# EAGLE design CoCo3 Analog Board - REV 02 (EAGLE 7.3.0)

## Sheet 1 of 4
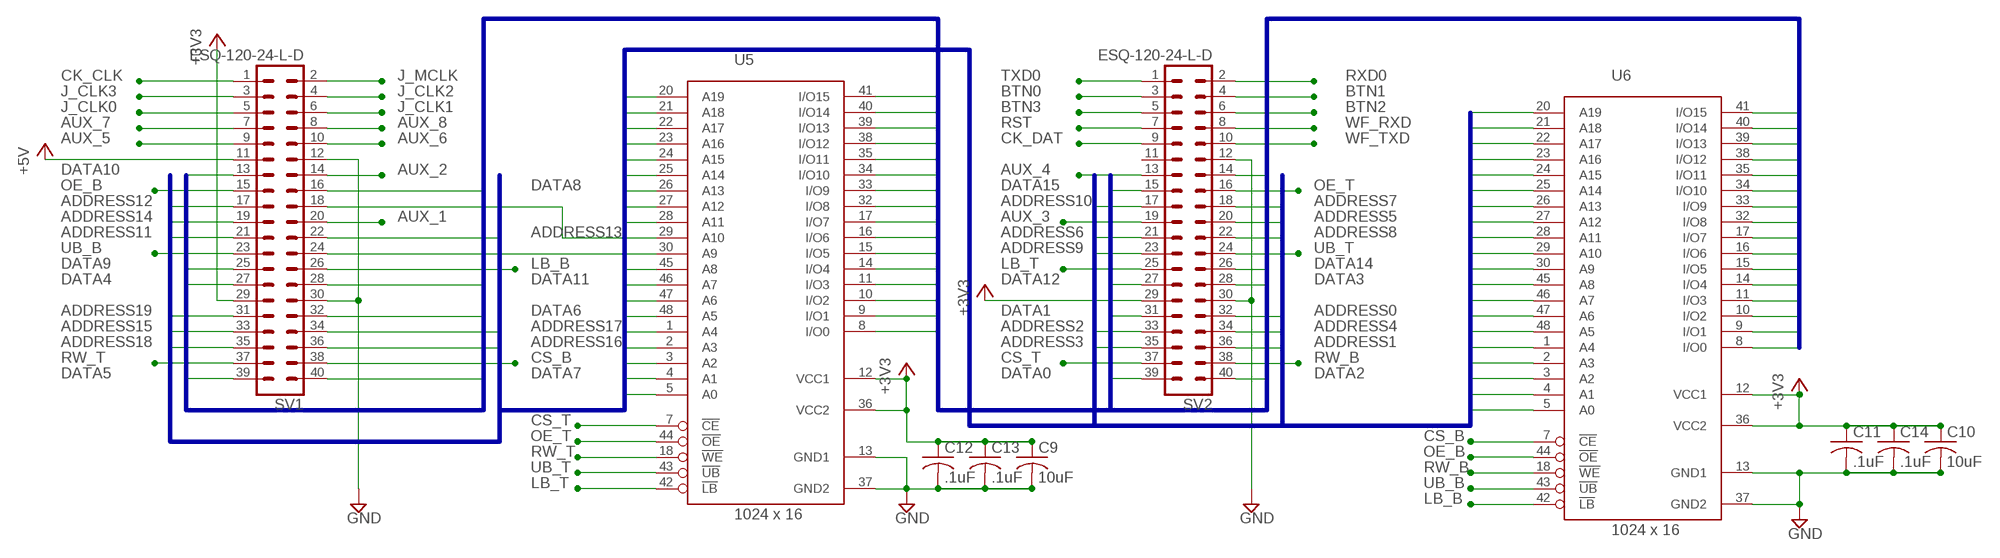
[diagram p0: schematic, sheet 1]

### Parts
C9  10uF  C-USC0805  [C0805]
C10  10uF  C-USC0805  [C0805]
C11  .1uF  C-USC0603  [C0603]
C12  .1uF  C-USC0603  [C0603]
C13  .1uF  C-USC0603  [C0603]
C14  .1uF  C-USC0603  [C0603]
SV1  ESQ-120-24-L-D  MA20-2  [MA20-2]
SV2  ESQ-120-24-L-D  MA20-2  [MA20-2]
U5  1024 x 16  IS62WV102416BLL-25T  [TSOP-I-48-12X40MM]
U6  1024 x 16  IS62WV102416BLL-25T  [TSOP-I-48-12X40MM]

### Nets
+3V3: C9.1 C10.1 C11.1 C12.1 C13.1 C14.1 SV1.29 SV2.29 U5.12(VCC1) U5.36(VCC2) U6.12(VCC1) U6.36(VCC2) ; also sheet 2,4
+5V: SV1.11 ; also sheet 3,4
ADDRESS0: SV2.32 U5.5(A0) U6.20(A19)
ADDRESS1: SV2.36 U5.4(A1) U6.21(A18)
ADDRESS2: SV2.33 U5.3(A2) U6.22(A17)
ADDRESS3: SV2.35 U5.2(A3) U6.23(A16)
ADDRESS4: SV2.34 U5.1(A4) U6.24(A15)
ADDRESS5: SV2.20 U5.48(A5) U6.25(A14)
ADDRESS6: SV2.21 U5.47(A6) U6.26(A13)
ADDRESS7: SV2.18 U5.46(A7) U6.27(A12)
ADDRESS8: SV2.22 U5.45(A8) U6.28(A11)
ADDRESS9: SV2.23 U6.30(A9)
ADDRESS9T: SV1.24 U5.30(A9)
ADDRESS10: SV2.17 U6.29(A10)
ADDRESS10T: SV1.18 U5.29(A10)
ADDRESS11: SV1.21 U5.28(A11) U6.45(A8)
ADDRESS12: SV1.17 U5.27(A12) U6.46(A7)
ADDRESS13: SV1.22 U5.26(A13) U6.47(A6)
ADDRESS14: SV1.19 U5.25(A14) U6.48(A5)
ADDRESS15: SV1.33 U5.24(A15) U6.1(A4)
ADDRESS16: SV1.36 U5.23(A16) U6.2(A3)
ADDRESS17: SV1.34 U5.22(A17) U6.3(A2)
ADDRESS18: SV1.35 U5.21(A18) U6.4(A1)
ADDRESS19: SV1.31 U5.20(A19) U6.5(A0)
AUX_1: SV1.20 ; also sheet 4
AUX_2: SV1.14 ; also sheet 4
AUX_3: SV2.19 ; also sheet 4
AUX_4: SV2.13 ; also sheet 4
AUX_5: SV1.9 ; also sheet 4
AUX_6: SV1.10 ; also sheet 4
AUX_7: SV1.7 ; also sheet 4
AUX_8: SV1.8 ; also sheet 4
BTN0: SV2.3 ; also sheet 3
BTN1: SV2.4 ; also sheet 3
BTN2: SV2.6 ; also sheet 3
BTN3: SV2.5 ; also sheet 3
CK_CLK: SV1.1 ; also sheet 4
CK_DAT: SV2.9 ; also sheet 4
CS_B: SV1.38 U6.7(!CE)
CS_T: SV2.37 U5.7(!CE)
DATA0: SV2.39 U5.8(I/O0) U6.17(I/O7)
DATA1: SV2.31 U5.9(I/O1) U6.16(I/O6)
DATA2: SV2.40 U5.10(I/O2) U6.15(I/O5)
DATA3: SV2.28 U5.11(I/O3) U6.14(I/O4)
DATA4: SV1.27 U5.14(I/O4) U6.11(I/O3)
DATA5: SV1.39 U5.15(I/O5) U6.10(I/O2)
DATA6: SV1.32 U5.16(I/O6) U6.9(I/O1)
DATA7: SV1.40 U5.17(I/O7) U6.8(I/O0)
DATA8: SV1.16 U5.32(I/O8) U6.41(I/O15)
DATA9: SV1.25 U5.33(I/O9) U6.40(I/O14)
DATA10: SV1.13 U5.34(I/O10) U6.39(I/O13)
DATA11: SV1.28 U5.35(I/O11) U6.38(I/O12)
DATA12: SV2.27 U5.38(I/O12) U6.35(I/O11)
DATA13: SV2.14 U5.39(I/O13) U6.34(I/O10)
DATA14: SV2.26 U5.40(I/O14) U6.33(I/O9)
DATA15: SV2.15 U5.41(I/O15) U6.32(I/O8)
GND: C9.2 C10.2 C11.2 C12.2 C13.2 C14.2 SV1.12 SV1.30 SV2.12 SV2.30 U5.13(GND1) U5.37(GND2) U6.13(GND1) U6.37(GND2) ; also sheet 2,3,4
J_CLK0: SV1.5 ; also sheet 3
J_CLK1: SV1.6 ; also sheet 3
J_CLK2: SV1.4 ; also sheet 3
J_CLK3: SV1.3 ; also sheet 3
J_MCLK: SV1.2 ; also sheet 3
LB_B: SV1.26 U6.42(!LB)
LB_T: SV2.25 U5.42(!LB)
OE_B: SV1.15 U6.44(!OE)
OE_T: SV2.16 U5.44(!OE)
RST: SV2.7 ; also sheet 4
RW_B: SV2.38 U6.18(!WE)
RW_T: SV1.37 U5.18(!WE)
RXD0: SV2.2 ; also sheet 2
TXD0: SV2.1 ; also sheet 2
UB_B: SV1.23 U6.43(!UB)
UB_T: SV2.24 U5.43(!UB)
WF_RXD: SV2.8 ; also sheet 4
WF_TXD: SV2.10 ; also sheet 4
Unconnected: SV2.11

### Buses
DATA[0..15]
ADDRESS[0..19]

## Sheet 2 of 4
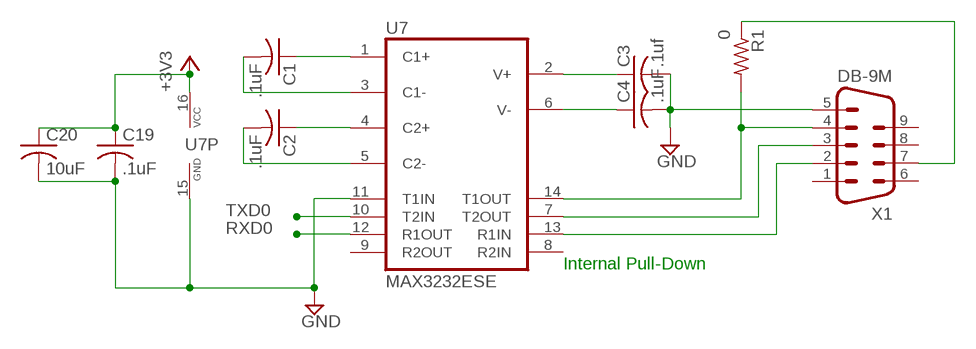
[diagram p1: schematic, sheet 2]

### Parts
C1  .1uF  C-USC0603  [C0603]
C2  .1uF  C-USC0603  [C0603]
C3  .1uf  C-USC0603  [C0603]
C4  .1uF  C-USC0603  [C0603]
C19  .1uF  C-USC0603  [C0603]
C20  10uF  C-USC0805  [C0805]
R1  0  R-US_M0805  [M0805]
U7  MAX3232ESE  [SO16]
X1  DB-9M  M09HP  [M09HP]

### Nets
+3V3: C19.1 C20.1 U7.16(VCC) ; also sheet 1,4
GND: C3.2 C4.2 C19.2 C20.2 U7.11(T1IN) U7.15(GND) X1.5 ; also sheet 1,3,4
N$1: C1.1 U7.1(C1+)
N$2: C1.2 U7.3(C1-)
N$3: C2.1 U7.4(C2+)
N$4: C2.2 U7.5(C2-)
N$5: C3.1 U7.2(V+)
N$6: C4.1 U7.6(V-)
N$8: U7.13(R1IN) X1.2
N$9: U7.7(T2OUT) X1.3
N$27: R1.1 X1.7
N$28: R1.2 U7.14(T1OUT) X1.4
RXD0: U7.12(R1OUT) ; also sheet 1
TXD0: U7.10(T2IN) ; also sheet 1
Unconnected: U7.8(R2IN) U7.9(R2OUT) X1.1 X1.6 X1.8 X1.9

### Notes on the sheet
- Internal Pull-Down

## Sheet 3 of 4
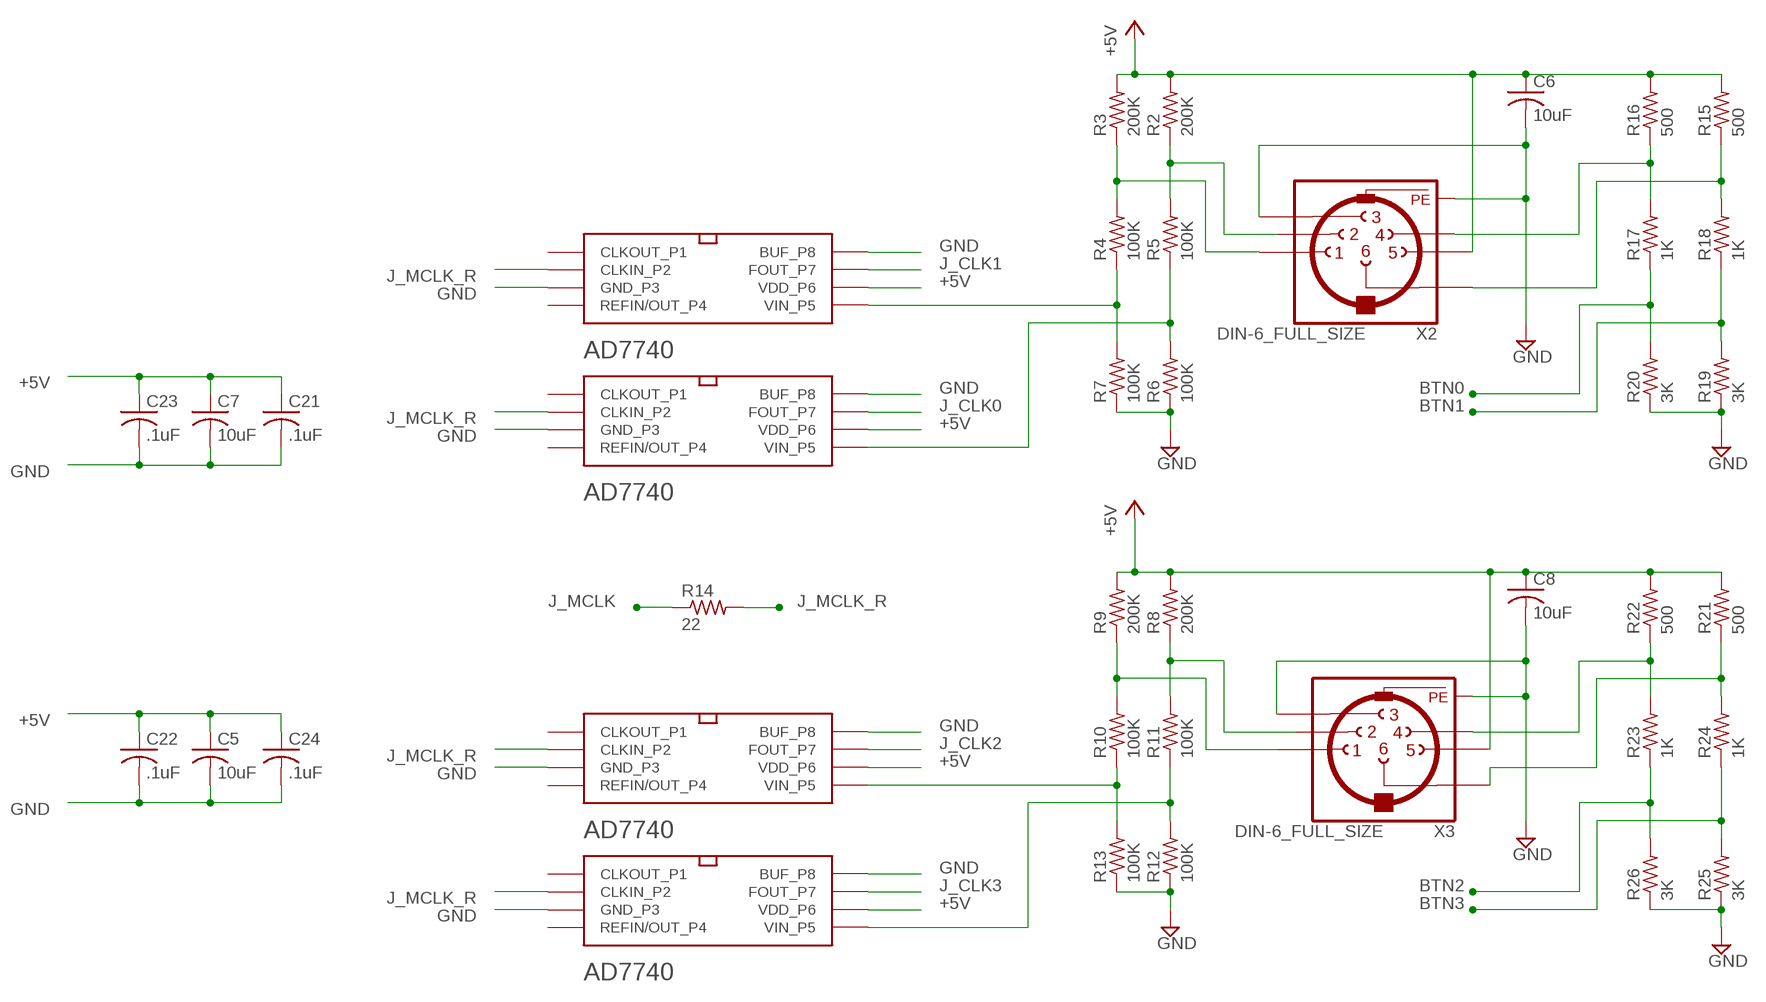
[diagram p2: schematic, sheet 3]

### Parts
C5  10uF  C-USC0805K  [C0805K]
C6  10uF  C-USC0805K  [C0805K]
C7  10uF  C-USC0805K  [C0805K]
C8  10uF  C-USC0805K  [C0805K]
C21  .1uF  C-USC0603  [C0603]
C22  .1uF  C-USC0603  [C0603]
C23  .1uF  C-USC0603  [C0603]
C24  .1uF  C-USC0603  [C0603]
R2  200K  R-US_M0805  [M0805]
R3  200K  R-US_M0805  [M0805]
R4  100K  R-US_M0805  [M0805]
R5  100K  R-US_M0805  [M0805]
R6  100K  R-US_M0805  [M0805]
R7  100K  R-US_M0805  [M0805]
R8  200K  R-US_M0805  [M0805]
R9  200K  R-US_M0805  [M0805]
R10  100K  R-US_M0805  [M0805]
R11  100K  R-US_M0805  [M0805]
R12  100K  R-US_M0805  [M0805]
R13  100K  R-US_M0805  [M0805]
R14  22  R-US_R0805  [R0805]
R15  500  R-US_R0805  [R0805]
R16  500  R-US_R0805  [R0805]
R17  1K  R-US_R0805  [R0805]
R18  1K  R-US_R0805  [R0805]
R19  3K  R-US_R0805  [R0805]
R20  3K  R-US_R0805  [R0805]
R21  500  R-US_R0805  [R0805]
R22  500  R-US_R0805  [R0805]
R23  1K  R-US_R0805  [R0805]
R24  1K  R-US_R0805  [R0805]
R25  3K  R-US_R0805  [R0805]
R26  3K  R-US_R0805  [R0805]
U$1  AD7740_MSOP-8  [AD7740_MSOP-8]
U$2  AD7740_MSOP-8  [AD7740_MSOP-8]
U$3  AD7740_MSOP-8  [AD7740_MSOP-8]
U$4  AD7740_MSOP-8  [AD7740_MSOP-8]
X2  DIN-6_FULL_SIZE  [DIN-6_FULL_SIZE]
X3  DIN-6_FULL_SIZE  [DIN-6_FULL_SIZE]

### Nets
+5V: C5.1 C6.1 C7.1 C8.1 C21.1 C22.1 C23.1 C24.1 R2.2 R3.2 R8.2 R9.2 R15.2 R16.2 R21.2 R22.2 U$1.P$06(VDD_P6) U$2.P$06(VDD_P6) U$3.P$06(VDD_P6) U$4.P$06(VDD_P6) X2.5 X3.5 ; also sheet 1,4
BTN0: R17.1 R20.2 ; also sheet 1
BTN1: R18.1 R19.2 ; also sheet 1
BTN2: R23.1 R26.2 ; also sheet 1
BTN3: R24.1 R25.2 ; also sheet 1
GND: C5.2 C6.2 C7.2 C8.2 C21.2 C22.2 C23.2 C24.2 R6.1 R7.1 R12.1 R13.1 R19.1 R20.1 R25.1 R26.1 U$1.P$3(GND_P3) U$1.P$08(BUF_P8) U$2.P$3(GND_P3) U$2.P$08(BUF_P8) U$3.P$3(GND_P3) U$3.P$08(BUF_P8) U$4.P$3(GND_P3) U$4.P$08(BUF_P8) X2.3 X2.PE X2.PE@(PE) X3.3 X3.PE X3.PE@(PE) ; also sheet 1,2,4
J_CLK0: U$1.P$07(FOUT_P7) ; also sheet 1
J_CLK1: U$2.P$07(FOUT_P7) ; also sheet 1
J_CLK2: U$4.P$07(FOUT_P7) ; also sheet 1
J_CLK3: U$3.P$07(FOUT_P7) ; also sheet 1
J_MCLK: R14.1 ; also sheet 1
J_MCLK_R: R14.2 U$1.P$2(CLKIN_P2) U$2.P$2(CLKIN_P2) U$3.P$2(CLKIN_P2) U$4.P$2(CLKIN_P2)
N$11: R22.1 R23.2 X3.4
N$12: R3.1 R4.2 X2.1
N$14: R5.1 R6.2 U$1.P$05(VIN_P5)
N$15: R2.1 R5.2 X2.2
N$16: R21.1 R24.2 X3.6
N$17: R9.1 R10.2 X3.1
N$18: R10.1 R13.2 U$4.P$05(VIN_P5)
N$19: R11.1 R12.2 U$3.P$05(VIN_P5)
N$20: R8.1 R11.2 X3.2
N$21: R16.1 R17.2 X2.4
N$22: R15.1 R18.2 X2.6
N$25: R4.1 R7.2 U$2.P$05(VIN_P5)
Unconnected: U$1.P$1(CLKOUT_P1) U$1.P$4(REFIN/OUT_P4) U$2.P$1(CLKOUT_P1) U$2.P$4(REFIN/OUT_P4) U$3.P$1(CLKOUT_P1) U$3.P$4(REFIN/OUT_P4) U$4.P$1(CLKOUT_P1) U$4.P$4(REFIN/OUT_P4)

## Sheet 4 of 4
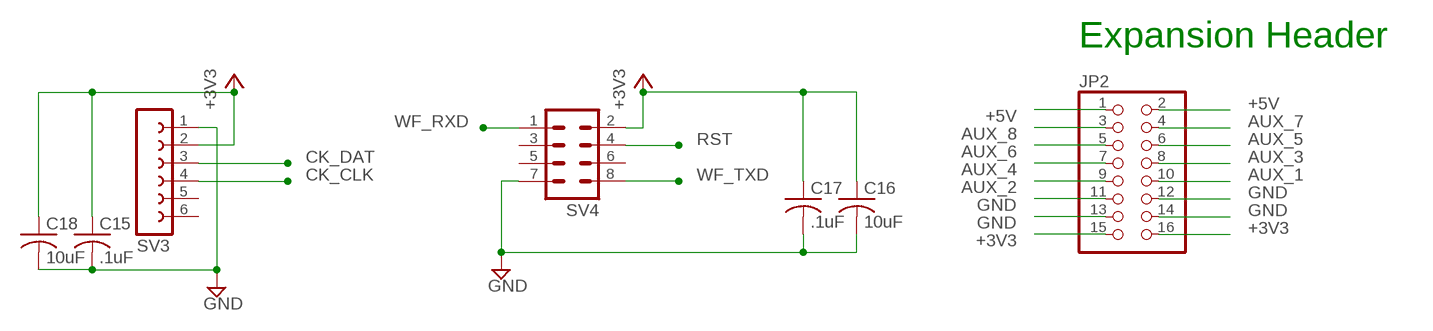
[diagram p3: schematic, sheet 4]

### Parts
C15  .1uF  C-USC0603  [C0603]
C16  10uF  C-USC0805  [C0805]
C17  .1uF  C-USC0603  [C0603]
C18  10uF  C-USC0805  [C0805]
JP2  PIN_HEADER_02X08  [PIN_HEADER_2X08]
SV3  FE06-1  [FE06]
SV4  MA04-2  [MA04-2]

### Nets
+3V3: C15.1 C16.1 C17.1 C18.1 JP2.15 JP2.16 SV3.2 SV4.2 ; also sheet 1,2
+5V: JP2.1 JP2.2 ; also sheet 1,3
AUX_1: JP2.10 ; also sheet 1
AUX_2: JP2.9 ; also sheet 1
AUX_3: JP2.8 ; also sheet 1
AUX_4: JP2.7 ; also sheet 1
AUX_5: JP2.6 ; also sheet 1
AUX_6: JP2.5 ; also sheet 1
AUX_7: JP2.4 ; also sheet 1
AUX_8: JP2.3 ; also sheet 1
CK_CLK: SV3.4 ; also sheet 1
CK_DAT: SV3.3 ; also sheet 1
GND: C15.2 C16.2 C17.2 C18.2 JP2.11 JP2.12 JP2.13 JP2.14 SV3.1 SV4.7 ; also sheet 1,2,3
RST: SV4.4 ; also sheet 1
WF_RXD: SV4.1 ; also sheet 1
WF_TXD: SV4.8 ; also sheet 1
Unconnected: SV3.5 SV3.6 SV4.3 SV4.5 SV4.6

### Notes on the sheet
- Expansion Header

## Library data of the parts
C1-C4 C11-C15 C17 C19 C21-C24 = resistor:C-US: CAPACITOR, American symbol
C5-C10 C16 C18 C20 = rcl:C-US: CAPACITOR, American symbol
JP2 = Zippster's Parts:PIN_HEADER_02X08: PIN HEADER
R1-R26 = rcl:R-US_: RESISTOR, American symbol
SV1 SV2 = con-lstb:MA20-2: PIN HEADER; OC_FARNELL: unknown; OC_NEWARK: unknown
SV3 = con-lsta:FE06-1: FEMALE HEADER; OC_FARNELL: unknown; OC_NEWARK: unknown
SV4 = con-lstb:MA04-2: PIN HEADER; OC_FARNELL: unknown; OC_NEWARK: unknown
U5 U6 = Gary_LBR:IS62WV102416BLL-*: 1024k x 16 high- speed low power CMOS static RAM 25ns access time 3.6V power supply
U7 = maxim:MAX3232*: True RS-232 Transceivers 3.0V to 5.5V, Low-Power up to 1Mbps, Using Four 0.1µF External Capacitors Source: http://pdfserv.maxim-ic.com/en/ds/MAX3222-MAX3241.pdf; MF: MAXIM; MPN: MAX3232ESE; OC_FARNELL: 9725539; OC_NEWARK: 79C3880
U$1-U$4 = Zippster's Parts:AD7740_MSOP-8
X1 = con-subd:M09: SUB-D; OC_FARNELL: unknown; OC_NEWARK: unknown
X2 X3 = Zippster's Parts:DIN-6_FULL_SIZE: Female CONNECTOR 6 pins with shield, horizontal (DIN 45322); MF: FARNELL; MPN: MAB 6 H; OC_FARNELL: 809901; OC_NEWARK: 67C7887

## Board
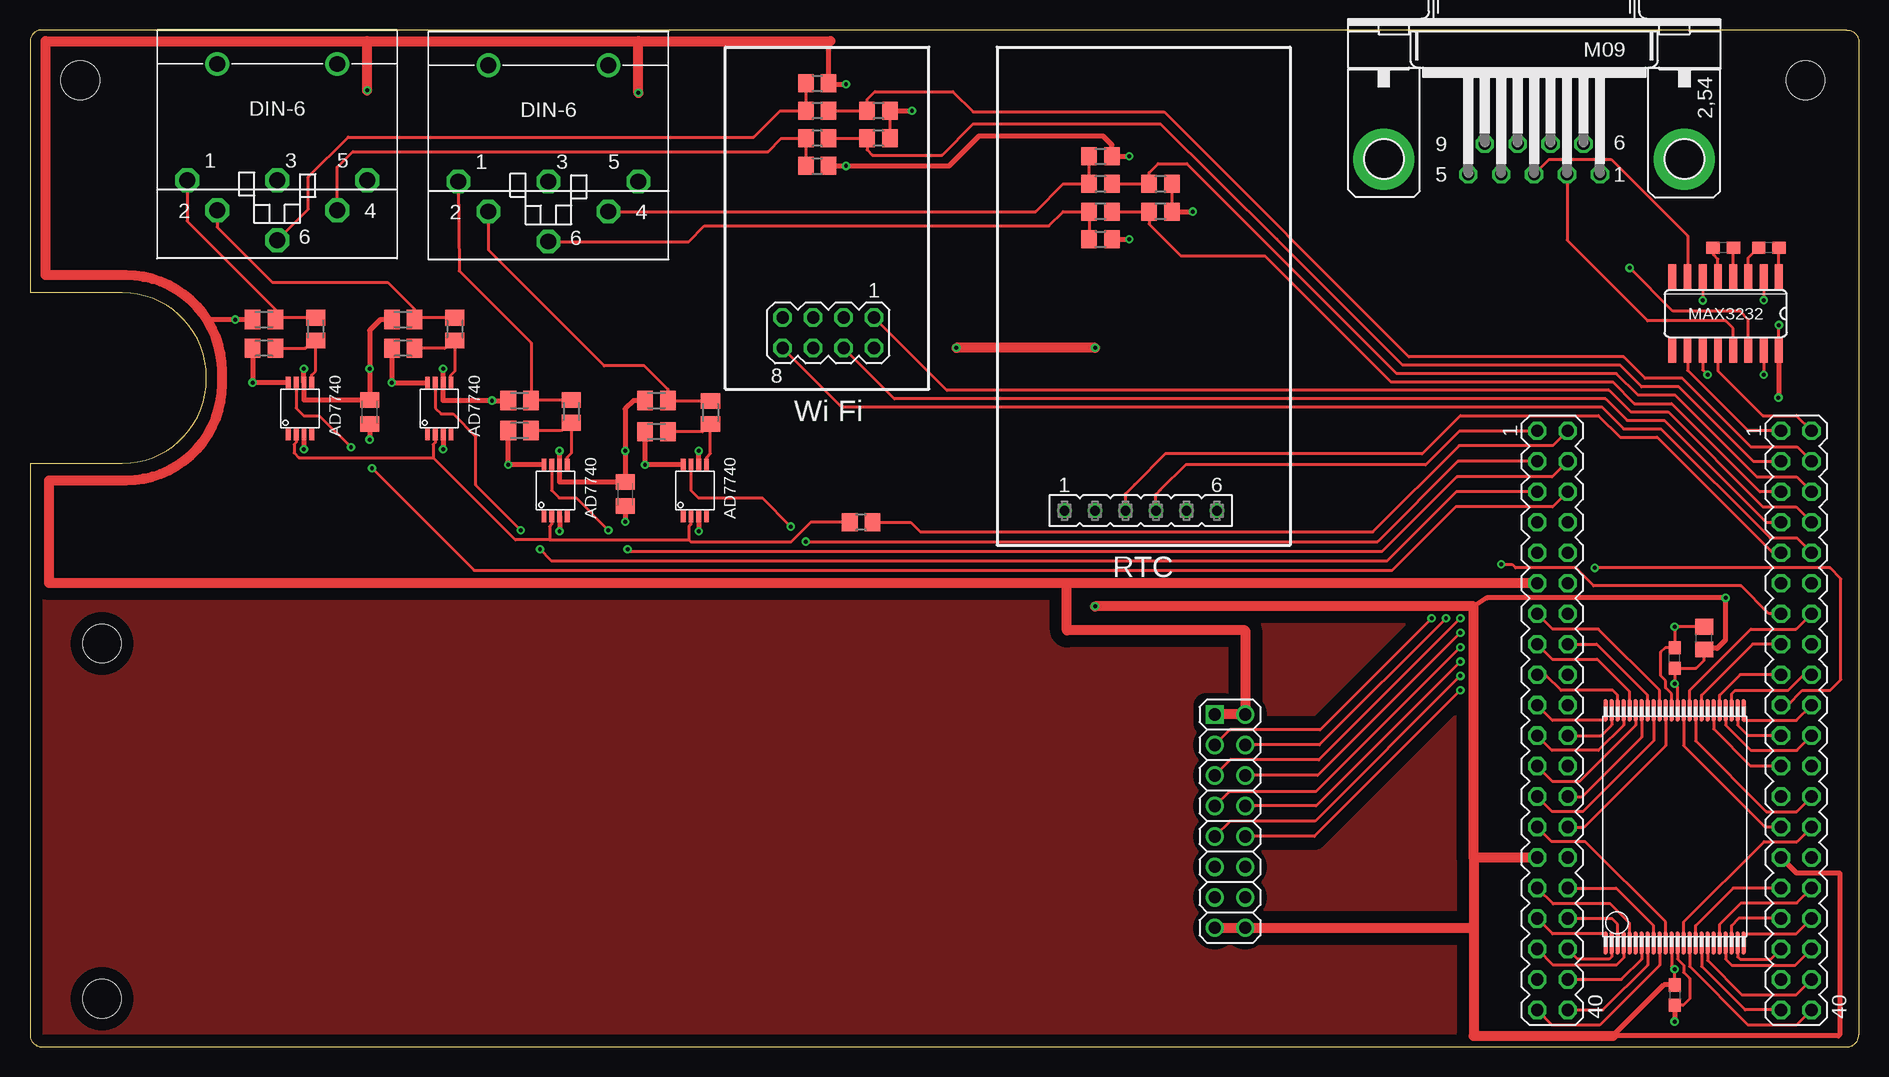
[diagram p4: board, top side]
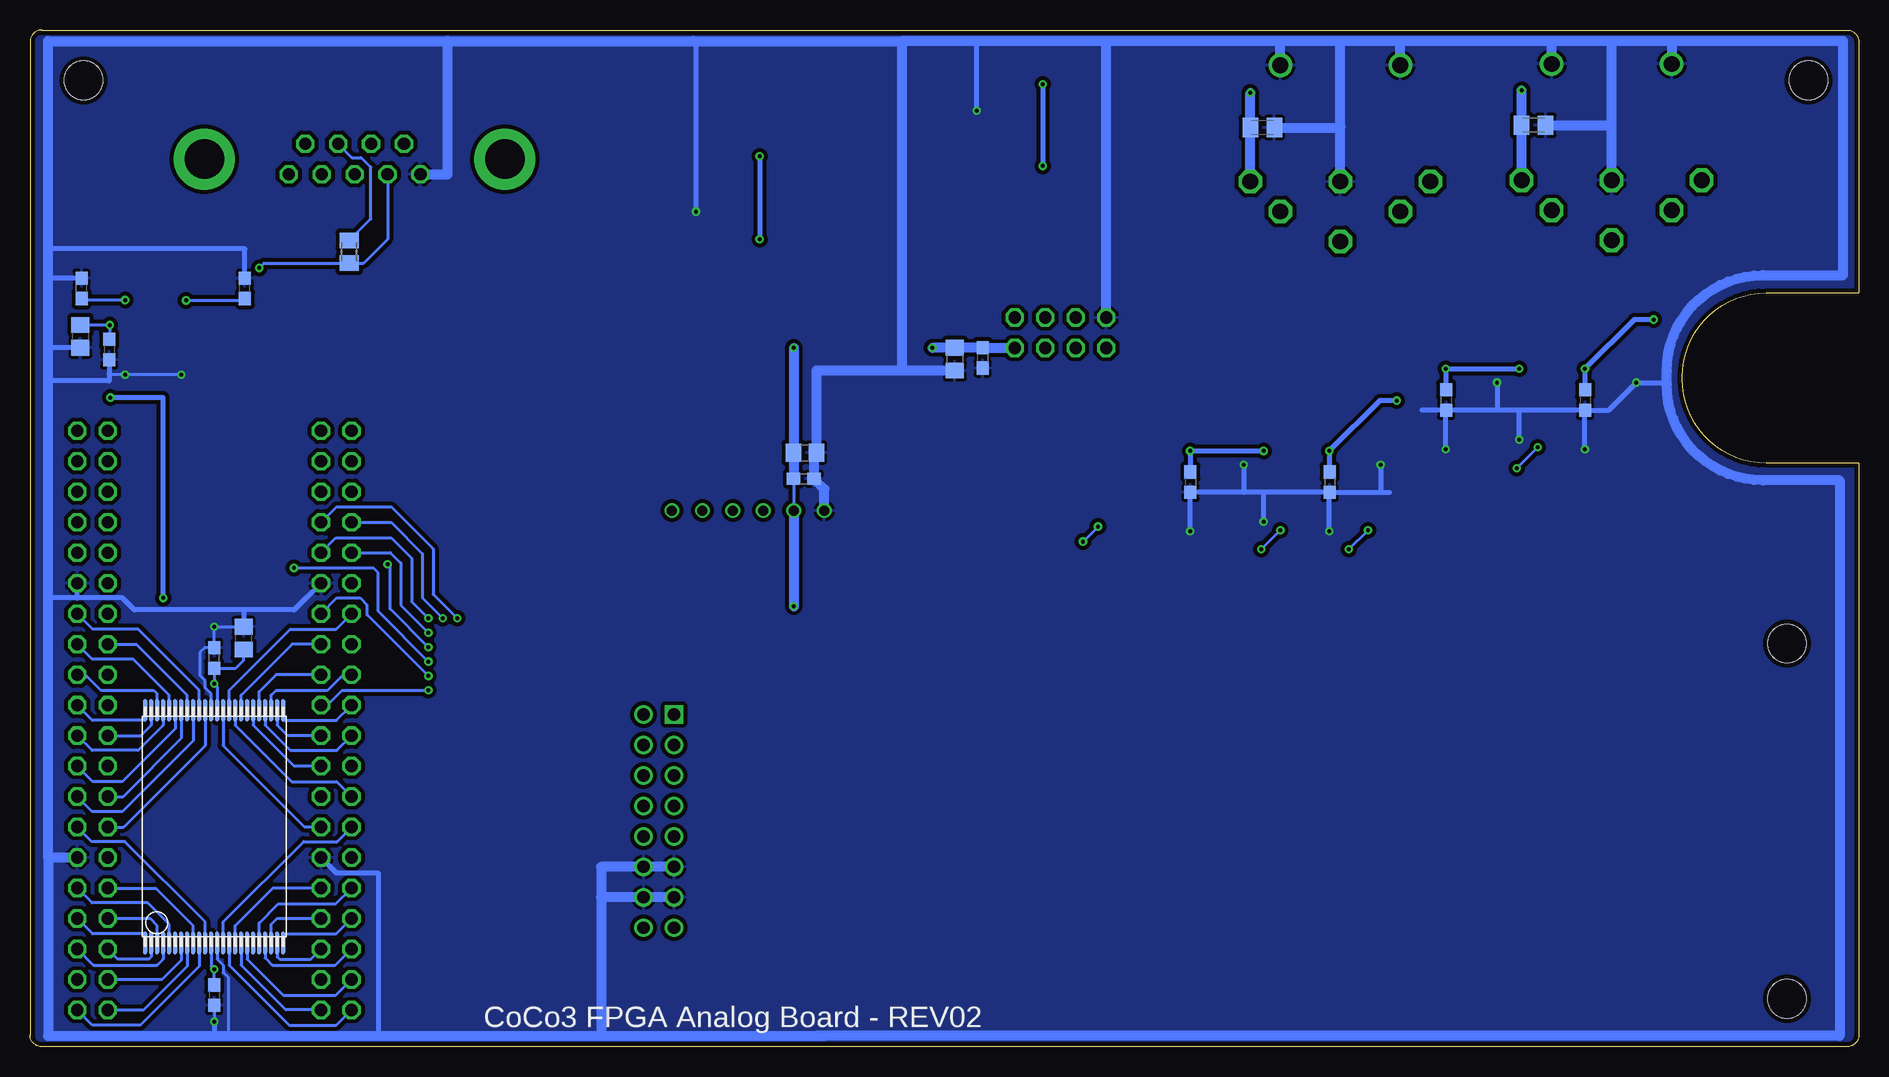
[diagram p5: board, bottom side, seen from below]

Size 152.4 x 84.73 mm. Coordinates in mm from the lower left corner, seen from the top.
Outline: 1,0 151.4,0 arc90 152.4,1 152.4,83.73 arc90 151.4,84.73 1,84.73 arc90 0,83.73 0,62.83 7.7,62.83 arc-90 14.7,55.83 14.7,55.63 arc-90 7.7,48.63 0,48.63 0,1 arc90 1,0
Copper layers (1*16): Top 0.0356mm / dielectric 1.5011mm / Bottom 0.0356mm
Design rules "LaenPCBOrder *": minimum track width 6mil, minimum drill 13mil, track to track 6mil, track to pad 6mil, pad to pad 6mil, via to via 6mil, smd to smd 6mil, copper to edge 15mil, drill to drill 6mil, minimum pad ring 7mil, minimum via ring 7mil, stop-mask expansion 3mil, vias tented up to drill 0.7mm, thermal gap 10mil
Holes 3.2 mm at 147.96,80.54 4.19,80.54 6,4 6,33.6

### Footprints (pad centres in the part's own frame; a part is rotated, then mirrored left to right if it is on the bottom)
C0603 = smd 1.1 x 1: 1 -0.85,0; 2 0.85,0
C0805K = smd 1.3 x 1.6: 1 -1,0; 2 1,0
C0805 = smd 1.3 x 1.5: 1 -0.95,0; 2 0.95,0
PIN_HEADER_2X08 = drill 1.016 square: 1 -8.89,-1.27 | drill 1.016: 2 -8.89,1.27; 3 -6.35,-1.27; 4 -6.35,1.27; 5 -3.81,-1.27; 6 -3.81,1.27; 7 -1.27,-1.27; 8 -1.27,1.27; 9 1.27,-1.27; 10 1.27,1.27; 11 3.81,-1.27; 12 3.81,1.27; 13 6.35,-1.27; 14 6.35,1.27; 15 8.89,-1.27; 16 8.89,1.27
M0805 = smd 1.3 x 1.6: 1 -0.95,0; 2 0.95,0
R0805 = smd 1.3 x 1.5: 1 -0.95,0; 2 0.95,0
MA20-2 = drill 1.016 octagon: 1 -24.13,-1.27; 2 -24.13,1.27; 3 -21.59,-1.27; 4 -21.59,1.27; 5 -19.05,-1.27; 6 -19.05,1.27; 7 -16.51,-1.27; 8 -16.51,1.27; 9 -13.97,-1.27; 10 -13.97,1.27; 11 -11.43,-1.27; 12 -11.43,1.27; 13 -8.89,-1.27; 14 -8.89,1.27; 15 -6.35,-1.27; 16 -6.35,1.27; 17 -3.81,-1.27; 18 -3.81,1.27; 19 -1.27,-1.27; 20 -1.27,1.27; 21 1.27,-1.27; 22 1.27,1.27; 23 3.81,-1.27; 24 3.81,1.27; 25 6.35,-1.27; 26 6.35,1.27; 27 8.89,-1.27; 28 8.89,1.27; 29 11.43,-1.27; 30 11.43,1.27; 31 13.97,-1.27; 32 13.97,1.27; 33 16.51,-1.27; 34 16.51,1.27; 35 19.05,-1.27; 36 19.05,1.27; 37 21.59,-1.27; 38 21.59,1.27; 39 24.13,-1.27; 40 24.13,1.27
FE06 = drill 0.813: 1 -6.35,0; 2 -3.81,0; 3 -1.27,0; 4 1.27,0; 5 3.81,0; 6 6.35,0
MA04-2 = drill 1.016 octagon: 1 -3.81,-1.27; 2 -3.81,1.27; 3 -1.27,-1.27; 4 -1.27,1.27; 5 1.27,-1.27; 6 1.27,1.27; 7 3.81,-1.27; 8 3.81,1.27
TSOP-I-48-12X40MM = smd 1.9 x 0.34: 1 -9.7,5.75; 2 -9.7,5.25; 3 -9.7,4.75; 4 -9.7,4.25; 5 -9.7,3.75; 6 -9.7,3.25; 7 -9.7,2.75; 8 -9.7,2.25; 9 -9.7,1.75; 10 -9.7,1.25; 11 -9.7,0.75; 12 -9.7,0.25; 13 -9.7,-0.25; 14 -9.7,-0.75; 15 -9.7,-1.25; 16 -9.7,-1.75; 17 -9.7,-2.25; 18 -9.7,-2.75; 19 -9.7,-3.25; 20 -9.7,-3.75; 21 -9.7,-4.25; 22 -9.7,-4.75; 23 -9.7,-5.25; 24 -9.7,-5.75; 25 9.7,-5.75; 26 9.7,-5.25; 27 9.7,-4.75; 28 9.7,-4.25; 29 9.7,-3.75; 30 9.7,-3.25; 31 9.7,-2.75; 32 9.7,-2.25; 33 9.7,-1.75; 34 9.7,-1.25; 35 9.7,-0.75; 36 9.7,-0.25; 37 9.7,0.25; 38 9.7,0.75; 39 9.7,1.25; 40 9.7,1.75; 41 9.7,2.25; 42 9.7,2.75; 43 9.7,3.25; 44 9.7,3.75; 45 9.7,4.25; 46 9.7,4.75; 47 9.7,5.25; 48 9.7,5.75
SO16 = smd 0.66 x 2.032: 1 -4.445,-3.073; 2 -3.175,-3.073; 3 -1.905,-3.073; 4 -0.635,-3.073; 5 0.635,-3.073; 6 1.905,-3.073; 7 3.175,-3.073; 8 4.445,-3.073; 9 4.445,3.073; 10 3.175,3.073; 11 1.905,3.073; 12 0.635,3.073; 13 -0.635,3.073; 14 -1.905,3.073; 15 -3.175,3.073; 16 -4.445,3.073
AD7740_MSOP-8 = smd 0.4 x 1: P$1 -0.975,-2.15; P$2 -0.325,-2.15; P$3 0.325,-2.15; P$4 0.975,-2.15; P$05 0.975,2.15; P$06 0.325,2.15; P$07 -0.325,2.15; P$08 -0.975,2.15
M09HP = drill 1.016 octagon: 1 -5.486,1.27; 2 -2.743,1.27; 3 0,1.27; 4 2.743,1.27; 5 5.486,1.27; 6 -4.115,-1.27; 7 -1.372,-1.27; 8 1.372,-1.27; 9 4.115,-1.27 | drill 3.302 pad 5.08: G1 -12.522,0; G2 12.522,0
DIN-6_FULL_SIZE = drill 1.321 octagon: 1 7.5,12.5; 2 5,15; 3 0,12.5; 4 -5,15; 5 -7.5,12.5; 6 0,17.5 | drill 1.321: PE -5,2.8; PE@ 5,2.8

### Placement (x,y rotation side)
C1  144.9,66.6 180 top
C2  141.1,66.6 180 top
C3  148.1,63.2 90 bottom
C4  134.5,63.2 90 bottom
C5  28.3,52.9 270 top
C6  27.1,76.8 0 bottom
C7  49.6,46.05 270 top
C8  49.7,76.6 0 bottom
C9  134.6,34.05 90 bottom
C10  139.5,34.05 90 top
C11  137.05,32.4 90 top
C12  137.05,32.4 90 bottom
C13  137.05,4.3 270 bottom
C14  137.05,4.3 270 top
C15  87.92,47.34 0 bottom
C16  75.33,57.3 270 bottom
C17  73.03,57.41 270 bottom
C18  87.83,49.51 0 bottom
C19  145.8,58.1 270 bottom
C20  148.2,59.2 270 bottom
C21  44.1,47.05 270 bottom
C22  55.7,47.05 270 bottom
C23  22.8,53.9 270 bottom
C24  34.4,53.9 270 bottom
JP2  100,18.8 270 top
R1  125.8,66.25 270 bottom
R2  31.1,60.6 180 top
R3  19.5,60.6 180 top
R4  23.8,59.8 90 top
R5  35.4,59.8 90 top
R6  31.1,58.2 0 top
R7  19.5,58.2 0 top
R8  52.2,53.85 180 top
R9  40.8,53.85 180 top
R10  45.1,52.95 90 top
R11  56.7,52.85 90 top
R12  52.2,51.25 0 top
R13  40.8,51.35 0 top
R14  69.26,43.71 180 top
R15  65.6,80.3 0 top
R16  65.6,73.4 0 top
R17  65.6,75.7 180 top
R18  65.6,78 180 top
R19  70.7,78 180 top
R20  70.7,75.7 180 top
R21  89.2,67.3 0 top
R22  89.2,74.2 0 top
R23  89.2,71.9 180 top
R24  89.2,69.6 180 top
R25  94.2,69.6 180 top
R26  94.2,71.9 180 top
SV1  126.87,27.2 270 top
SV2  147.19,27.2 270 top
SV3  92.56,44.67 0 top
SV4  66.53,59.5 180 top
U5  137.05,18.35 90 bottom
U6  137.05,18.35 90 top
U7  141.3,61.1 180 top
U$1  34.1,53.2 0 top
U$2  22.5,53.2 0 top
U$3  55.4,46.35 0 top
U$4  43.8,46.35 0 top
X1  125.34,73.97 180 top
X2  20.6,84.7 180 top
X3  43.2,84.6 180 top

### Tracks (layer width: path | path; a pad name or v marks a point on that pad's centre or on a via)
+3V3  (via drill 0.33)
  Top 0.254: U6.12 136.8,6.7 v137.05,6.45 C13.1 | U6.36 137.3,30 v137.05,30.25 C12.1 138.85,31.55 139.5,32.2 C10.1 | U7.16 v145.75,60.15
  Top 0.406: 131.9,0.9 136.15,5.15 C13.1 | SV2.29 147.19,14.5 150.8,14.5 150.8,1 150.7,0.9 127.4,0.9 | C10.1 139.6,33.2 140.6,33.2 141.3,33.9 v141.3,37.4 121.4,37.4 120.3,36.7 | U7.16 145.75,54.1 v145.7,54.1
  Top 0.813: SV1.29 120.3,15.77 | 120.3,15.77 120.3,9.91 | 120.3,9.91 120.3,0.9 127.4,0.9 131.9,0.9 | 120.3,15.77 120.3,36.7 v88.75,36.7 | v88.75,58.25 v77.2,58.25 | JP2.15 JP2.16 120.3,9.91
  Bottom 0.254: U5.12 137.3,6.7 v137.05,6.45 C13.1 | U5.36 136.8,30 v137.05,30.25 C12.1 135.25,31.55 134.6,32.2 C9.1 | C15.1 88.75,48.84 SV3.2 | C19.1 145.75,59.01 v145.75,60.15 147.59,60.15 C20.1
  Bottom 0.406: v141.3,37.4 141.3,54.1 v145.7,54.1
  Bottom 0.813: C15.1 C18.1 88.75,49.53 v88.75,58.25 | SV3.2 v88.75,36.7 | SV4.2 72.99,58.23 C17.1 75.31,58.26 C16.1 v77.2,58.25
+5V  (via drill 0.33)
  Top 0.254: 15,60.6 14.9,60.5 | 14.9,60.5 14.8,60.5 14.7,60.6 | 14.9,60.5 arc-90 15.2,60.2 15.2,59.5 arc-90 15.6,59.1 15.6,58.5 arc-90 15.9,58.2 15.9,57.4 arc-90 16,57.3 16,56.3 | 34.4,55.33 U$1.P$06
  Top 0.406: R3.2 v17.1,60.6 15,60.6 | v34.42,56.5 U$1.P$06 34.42,53.85 v38.5,53.85 R9.2 | v22.82,56.5 U$2.P$06 22.82,53.9 C5.1 v28.3,56.5 28.3,59.7 29.2,60.6 R2.2 | v44.12,49.65 U$4.P$06 44.12,47.05 C7.1 v49.6,49.65 49.6,53.15 50.3,53.85 R8.2 | U$3.P$06 v55.73,49.65 | 66.7,83.8 66.55,83.8 R15.2 66.55,80.2 v68,80.2 | R16.2 v68,73.4 76.6,73.4 79.1,75.9 89.4,75.9 90.15,75.15 R22.2 v91.6,74.2 | R21.2 v91.6,67.3
  Top 0.813: SV1.11 86.4,38.63 | 86.4,38.63 1.6,38.63 1.6,47.2 8,47.2 arc90 16,55.2 16,56.3 arc90 8,64.3 1.3,64.3 1.3,83.8 28.1,83.8 | 28.1,83.8 50.7,83.8 | v50.7,79.5 50.7,83.8 | v28.1,79.7 28.1,83.8 | 50.7,83.8 66.7,83.8 | JP2.1 JP2.2 101.27,34.7 86.4,34.7 86.4,38.63
  Bottom 0.406: C24.1 34.42,54.75 v34.42,56.5 v28.3,56.5 | C23.1 22.82,54.75 v22.82,56.5 18.73,60.6 v17.1,60.6 | C21.1 44.12,47.9 v44.12,49.65 39.92,53.85 v38.5,53.85 | C22.1 55.73,47.9 v55.73,49.65 v49.6,49.65 | v68,80.2 v68,73.4 | v91.6,74.2 v91.6,67.3
  Bottom 0.813: X3.5 C8.1 v50.7,79.5 | X2.5 C6.1 v28.1,79.7
ADDRESS0
  Top 0.254: U6.20 140.8,10.2 142.6,12 147.23,12 SV2.32
  Bottom 0.254: U6.20 140.8,10.2 142.6,12 147.23,12 SV2.32
ADDRESS1
  Top 0.254: U6.21 141.3,7.3 141.8,6.8 147.11,6.8 SV2.36
  Bottom 0.254: U6.21 141.3,7.3 141.8,6.8 147.11,6.8 SV2.36
ADDRESS2
  Top 0.254: U6.22 141.8,10.1 142.39,10.69 SV2.33
  Bottom 0.254: U6.22 141.8,10.1 142.39,10.69 SV2.33
ADDRESS3
  Top 0.254: U6.23 142.3,7.5 142.5,7.3 145.07,7.3 SV2.35
  Bottom 0.254: U6.23 142.3,7.5 142.5,7.3 145.07,7.3 SV2.35
ADDRESS4
  Top 0.254: U6.24 142.8,9.4 147.17,9.4 SV2.34
  Bottom 0.254: U6.24 142.8,9.4 147.17,9.4 SV2.34
ADDRESS5
  Top 0.254: U6.25 142.8,27.2 147.2,27.2 147.2,27.21 SV2.20
  Bottom 0.254: U6.25 142.8,27.2 147.19,27.2 SV2.20
ADDRESS6
  Top 0.254: U6.26 142.3,26.8 143.17,25.93 SV2.21
  Bottom 0.254: U6.26 142.3,26.8 143.17,25.93 SV2.21
ADDRESS7
  Top 0.254: U6.27 141.8,29.4 142.1,29.7 146.5,29.7 147.81,31.01 SV2.18
  Bottom 0.254: U6.27 141.8,29.4 142.1,29.7 146.5,29.7 147.81,31.01 SV2.18
ADDRESS8
  Top 0.254: U6.28 141.3,26.8 143.4,24.7 147.23,24.7 SV2.22
  Bottom 0.254: U6.28 141.3,26.8 143.4,24.7 147.23,24.7 SV2.22
ADDRESS9
  Top 0.254: U6.30 140.3,26.5 143.41,23.39 SV2.23
ADDRESS9T
  Bottom 0.254: U5.30 133.8,26.8 130.39,23.39 SV1.24
ADDRESS10
  Top 0.254: U6.29 140.8,29.3 142.51,31.01 SV2.17
ADDRESS10T
  Bottom 0.254: U5.29 133.3,29.6 131.89,31.01 SV1.18
ADDRESS11
  Top 0.254: U6.45 132.8,26.8 130.7,24.7 126.83,24.7 SV1.21
  Bottom 0.254: U6.45 132.8,26.8 130.7,24.7 126.83,24.7 SV1.21
ADDRESS12
  Top 0.254: U6.46 132.3,29.3 131.9,29.7 127.6,29.7 126.29,31.01 SV1.17
  Bottom 0.254: U6.46 132.3,29.3 131.9,29.7 127.6,29.7 126.29,31.01 SV1.17
ADDRESS13
  Top 0.254: U6.47 131.8,26.8 130.93,25.93 SV1.22
  Bottom 0.254: U6.47 131.8,26.8 130.93,25.93 SV1.22
ADDRESS14
  Top 0.254: U6.48 131.3,27.2 126.87,27.2 SV1.19
  Bottom 0.254: U6.48 131.3,27.2 126.87,27.2 SV1.19
ADDRESS15
  Top 0.254: U6.1 131.3,9.4 126.89,9.4 SV1.33
  Bottom 0.254: U6.1 131.3,9.4 126.89,9.4 SV1.33
ADDRESS16
  Top 0.254: U6.2 131.8,7.5 131.6,7.3 128.99,7.3 SV1.36
  Bottom 0.254: U6.2 131.8,7.5 131.6,7.3 128.99,7.3 SV1.36
ADDRESS17
  Top 0.254: U6.3 132.3,10.2 131.8,10.7 128.15,10.7 SV1.34
  Bottom 0.254: U6.3 132.3,10.2 131.8,10.7 128.15,10.7 SV1.34
ADDRESS18
  Top 0.254: U6.4 132.8,7.4 132.2,6.8 126.95,6.8 SV1.35
  Bottom 0.254: U6.4 132.8,7.4 132.2,6.8 126.95,6.8 SV1.35
ADDRESS19
  Top 0.254: U6.5 133.3,10.3 131.7,11.9 126.93,11.9 SV1.31
  Bottom 0.254: U6.5 133.3,10.3 131.7,11.9 126.93,11.9 SV1.31
AUX_1  (via drill 0.33)
  Top 0.254: v119.2,29.7 107.03,17.53 JP2.10
  Bottom 0.254: SV1.20 127.63,28.47 126.4,29.7 v119.2,29.7
AUX_2  (via drill 0.33)
  Top 0.254: v119.2,30.9 107.1,18.8 100,18.8 JP2.9
  Bottom 0.254: SV1.14 126.83,37.4 124.9,37.4 124.3,36.8 124.3,36 v119.2,30.9
AUX_3  (via drill 0.33)
  Top 0.254: SV2.19 146.47,28.47 147.7,29.7 150,29.7 150.9,30.6 150.9,39 150,39.9 v130.4,39.9 | v119.2,32.1 107.17,20.07 JP2.8
  Bottom 0.254: v130.4,39.9 123.8,39.9 123.4,39.5 123.4,36.3 v119.2,32.1
AUX_4  (via drill 0.33)
  Top 0.254: SV2.13 144.91,36.09 142.6,38.4 130.3,38.4 128.8,39.9 123.8,39.9 123.5,40.2 v122.6,40.2 | v119.2,33.3 107.2,21.3 99.96,21.3 JP2.7
  Bottom 0.254: v119.2,33.3 122.4,36.5 122.4,40 v122.6,40.2
AUX_5  (via drill 0.33)
  Top 0.254: v119.2,34.5 107.31,22.61 JP2.6
  Bottom 0.254: SV1.9 122.37,41.17 121.5,40.3 121.5,36.8 v119.2,34.5
AUX_6  (via drill 0.33)
  Top 0.254: v119.2,35.7 107.4,23.9 100.02,23.9 JP2.5
  Bottom 0.254: SV1.10 126.91,42.4 122.3,42.4 120.6,40.7 120.6,37.1 v119.2,35.7
AUX_7  (via drill 0.33)
  Top 0.254: v118,35.7 107.45,25.15 JP2.4
  Bottom 0.254: SV1.7 122.31,43.71 119.7,41.1 119.7,37.4 v118,35.7
AUX_8  (via drill 0.33)
  Top 0.254: v116.8,35.7 107.5,26.4 99.98,26.4 JP2.3
  Bottom 0.254: SV1.8 126.85,45 122.3,45 118.8,41.5 118.8,37.7 v116.8,35.7
BTN0
  Top 0.254: R17.1 R20.2 69.75,74.75 70.2,74.3 76,74.3 78.6,76.9 94.2,76.9 103.9,67.3 114.4,56.8 132.5,56.8 134.3,55 137.4,55 143.6,48.8 SV2.3
BTN1
  Top 0.254: R18.1 R19.2 69.75,78.95 70.4,79.6 76.9,79.6 78.6,77.9 94.5,77.9 114.9,57.5 132.8,57.5 134.6,55.7 137.7,55.7 143.4,50 147.25,50 SV2.4
BTN2
  Top 0.254: R23.1 R26.2 93.25,72.85 94,73.6 96.4,73.6 113.9,56.1 132.2,56.1 134,54.3 137.1,54.3 143.9,47.5 147.21,47.5 SV2.6
BTN3
  Top 0.254: R24.1 R25.2 93.25,68.55 95.9,65.9 102.9,65.9 113.4,55.4 131.9,55.4 133.7,53.6 136.8,53.6 144.15,46.25 SV2.5
CK_CLK
  Top 0.254: SV1.1 119.13,51.33 116.3,48.5 96.3,48.5 94.2,46.4 93.85,46.05 93.83,46.03 SV3.4
CK_DAT
  Top 0.254: SV2.9 145.23,41.17 135.6,50.8 132.5,50.8 130.7,52.6 119.2,52.6 116,49.4 94.6,49.4 92.05,46.85 91.3,46.1 91.29,46.09 SV3.3
CS_B
  Top 0.254: U6.7 134.3,7.3 132.61,5.61 SV1.38
CS_T
  Bottom 0.254: U5.7 139.8,7.2 141.39,5.61 SV2.37
DATA0
  Top 0.254: U6.17 139.3,6.7 142.93,3.07 SV2.39
  Bottom 0.254: U6.17 139.3,6.7 142.93,3.07 SV2.39
DATA1
  Top 0.254: U6.16 138.8,10.1 141.93,13.23 SV2.31
  Bottom 0.254: U6.16 138.8,10.1 141.93,13.23 SV2.31
DATA2
  Top 0.254: U6.15 138.3,6.7 143.2,1.8 147.19,1.8 SV2.40
  Bottom 0.254: SV2.40 147.19,1.8 143.2,1.8 138.3,6.7 U6.15
DATA3
  Top 0.254: U6.14 137.8,10.4 144.5,17.1 147.25,17.1 SV2.28
  Bottom 0.254: U6.14 137.8,10.4 144.5,17.1 147.25,17.1 SV2.28
DATA4
  Top 0.254: U6.11 136.3,10.4 129.6,17.1 126.81,17.1 | 126.81,17.1 126.8,17.1 | SV1.27 126.81,17.1
  Bottom 0.254: U6.11 136.3,10.4 129.6,17.1 126.81,17.1 SV1.27
DATA5
  Top 0.254: U6.10 135.8,6.8 130.8,1.8 126.87,1.8 SV1.39
  Bottom 0.254: U6.10 135.8,6.8 130.8,1.8 126.87,1.8 SV1.39
DATA6
  Top 0.254: U6.9 135.3,10.1 132.17,13.23 SV1.32
  Bottom 0.254: U6.9 135.3,10.1 132.17,13.23 SV1.32
DATA7
  Top 0.254: U6.8 134.8,6.8 131.07,3.07 SV1.40
  Bottom 0.254: U6.8 134.8,6.8 131.07,3.07 SV1.40
DATA8
  Top 0.254: U6.41 134.8,29.3 130.55,33.55 SV1.16
  Bottom 0.254: U6.41 134.8,29.3 130.55,33.55 SV1.16
DATA9
  Top 0.254: U6.40 135.3,25.5 129.4,19.6 126.85,19.6 SV1.25
  Bottom 0.254: U6.40 135.3,26.8 130.6,22.1 126.85,22.1 SV1.25
DATA10
  Top 0.254: U6.39 135.8,29.7 130.7,34.8 126.89,34.8 SV1.13
  Bottom 0.254: U6.39 135.8,29.7 130.7,34.8 126.89,34.8 SV1.13
DATA11
  Top 0.254: U6.38 136.3,25.1 129.51,18.31 | 129.51,18.31 129.5,18.3 | SV1.28 129.51,18.31
  Bottom 0.254: U6.38 136.3,25.1 129.51,18.31 SV1.28
DATA12
  Top 0.254: U6.35 137.8,25.1 144.59,18.31 SV2.27
  Bottom 0.254: U6.35 137.8,25.1 144.59,18.31 SV2.27
DATA13
  Top 0.254: U6.34 138.3,29.7 143.4,34.8 147.17,34.8 SV2.14
  Bottom 0.254: U6.34 138.3,29.7 143.4,34.8 147.17,34.8 SV2.14
DATA14
  Top 0.254: U6.33 138.8,25.5 144.7,19.6 147.21,19.6 SV2.26
  Bottom 0.254: U6.33 138.8,25.5 144.7,19.6 147.21,19.6 SV2.26
DATA15
  Top 0.254: U6.32 139.3,29.3 143.55,33.55 SV2.15
  Bottom 0.254: U6.32 139.3,29.3 143.55,33.55 SV2.15
GND  (via drill 0.33)
  Top 0.254: U6.13 137.3,7.3 137.8,6.8 137.8,6.2 138.3,5.7 138.3,4 137.75,3.45 C13.2 | U6.37 136.8,29.4 136.3,29.9 136.3,30.5 135.9,30.9 135.9,32.9 136.25,33.25 C12.2 v137.05,35 C10.2 | R26.1 R25.1 | R19.1 R20.1 | U7.11 139.4,56.41 v139.8,56 | U7.15 v144.47,56
  Top 0.406: C13.2 v137.05,2.1 | U$2.P$08 v18.55,55.35 R7.1 | R6.1 v30.15,55.35 U$1.P$08 | U$2.P$3 v22.82,49.8 | U$1.P$3 v34.42,49.8 | U$4.P$3 v44.12,42.95 | U$3.P$3 v55.73,42.95 | U$4.P$08 v39.85,48.5 R13.1 | C5.2 v28.3,50.6 | C7.2 v49.6,43.75 | U$3.P$08 v51.25,48.5 R12.1 | R19.1 v73.5,78 | R25.1 v96.9,69.6
  Bottom 0.254: U5.13 136.8,7.3 136.3,6.8 136.3,6.2 135.9,5.8 135.9,0.9 | C13.2 137.05,1.1 | U5.37 137.3,29.4 137.8,29.9 137.8,30.5 138.2,30.9 138.2,32.9 137.85,33.25 C12.2 v137.05,35 C9.2 | C18.2 87.08,49.71 | 16,55.35 16,55.2 | v139.8,56 v144.47,56 145.7,56 145.8,56.1
  Bottom 0.406: v137.05,2.1 137.05,1.1 137.05,0.9 136.9,0.9 | SV1.30 126.87,14.5 123.4,14.5 123.4,0.9 | 134.6,36.4 C9.2 | 148.46,37.4 144.7,37.4 143.7,36.4 134.6,36.4 | 148.46,37.4 SV2.12 | 16,55.35 v18.55,55.35 20.85,53.05 C23.2 | C23.2 28.3,53.05 | 28.3,53.05 30.15,53.05 | 30.15,53.05 C24.2 | v30.15,55.35 30.15,53.05 | C21.2 49.6,46.2 | 49.6,46.2 51.25,46.2 | 51.25,46.2 C22.2 55.73,46.17 v55.73,42.95 | v22.82,49.8 22.82,53.05 C23.2 | v34.42,49.8 34.42,53.05 C24.2 | v44.12,42.95 44.12,46.17 C21.2 | v28.3,50.6 28.3,53.05 | v49.6,43.75 49.6,46.2 | v51.25,48.5 51.25,46.2 | C24.2 36.4,53.05 | C21.2 39.8,46.2 | 39.8,46.2 39.1,46.2 | v39.85,48.5 39.85,46.25 39.8,46.2 | v73.5,78 73.5,83.8 72.3,83.8 | v96.9,69.6 96.9,83.8 97.1,83.8 | 148.46,37.4 150.9,37.4 | SV1.12 129.37,37.4 129.4,37.4 130.4,36.4 134.6,36.4 | C3.2 150.9,64.05 150.9,64 | C20.2 150.9,58.25 150.9,58.2 | C19.2 145.8,56.1 145.8,55.5 150.9,55.5 | C4.2 134.5,66.5 150.9,66.5
  Bottom 0.813: SV2.30 150.9,15.77 | 150.9,15.77 150.9,0.9 136.9,0.9 135.9,0.9 123.4,0.9 104.8,0.9 | 87.08,49.71 C15.2 86.21,46.48 SV3.1 | 104.8,0.9 86.21,0.9 | 86.9,0.9 1.6,0.9 1.6,47.2 8,47.2 arc90 16,55.2 16,56.3 arc90 8,64.3 1.3,64.3 1.3,83.8 15.6,83.8 | 15.6,83.8 X2.PE@ | 15.6,83.8 20.6,83.8 | 20.6,83.8 25.6,83.8 | 25.6,83.8 38.2,83.8 | 38.2,83.8 43.2,83.8 | 43.2,83.8 48.2,83.8 | 48.2,83.8 62.72,83.8 | 62.72,83.8 72.3,83.8 79.7,83.8 | X2.PE 25.6,83.8 | X3.PE@ 38.2,83.8 | X3.PE 48.2,83.8 | X2.3 20.6,76.8 | 20.6,76.8 20.6,83.8 | X3.3 43.2,76.7 | 43.2,76.7 43.2,83.8 | SV4.7 62.72,83.8 | C16.2 79.7,56.35 | 79.7,56.35 79.7,83.8 | 150.9,15.77 150.9,37.4 150.9,55.5 150.9,58.2 150.9,64 150.9,66.5 150.9,83.8 117.6,83.8 | 117.6,83.8 97.1,83.8 79.7,83.8 | C8.2 43.3,76.6 43.2,76.7 | C6.2 20.6,76.8 | 79.7,56.35 86.88,56.35 C18.2 | JP2.11 JP2.12 104.8,14.99 104.8,12.45 | JP2.13 JP2.14 104.8,12.45 | 104.8,12.45 104.8,0.9 | X1.5 117.6,72.7 117.6,83.8
  pour Bottom (isolate 0.33): 0.9,84.7 arc90 0,83.8 0,1 arc90 1,0 151.3,0 151.4,0 arc90 152.4,1 152.4,83.6 152.4,83.7 arc90 151.4,84.7
J_CLK0  (via drill 0.33)
  Top 0.254: U$1.P$07 33.77,53.23 34.25,52.75 35.25,52.75 37.15,50.85 37.15,46.8 v40.9,43.05 | SV1.5 118.85,46.25 113.1,40.5 43.45,40.5 v42.5,41.45
  Bottom 0.254: v42.5,41.45 v40.9,43.05
J_CLK1  (via drill 0.33)
  Top 0.254: U$2.P$07 22.18,53.23 22.8,52.6 24.1,52.6 v26.75,49.95 | SV1.6 126.89,45 118.8,45 113.5,39.7 37,39.7 v28.5,48.2
  Bottom 0.254: v26.75,49.95 v28.5,48.2
J_CLK2  (via drill 0.33)
  Top 0.254: U$4.P$07 43.48,46.38 44.1,45.75 45.5,45.75 v48.2,43.05 | SV1.4 126.85,47.5 118.9,47.5 112.7,41.3 49.95,41.3 v49.8,41.45
  Bottom 0.254: v48.2,43.05 v49.8,41.45
J_CLK3  (via drill 0.33)
  Top 0.254: U$3.P$07 55.08,46.38 55.7,45.75 61,45.75 v63.4,43.35 | v64.65,42.1 112.3,42.1 118.99,48.79 SV1.3
  Bottom 0.254: v64.65,42.1 v63.4,43.35
J_MCLK
  Top 0.254: R14.1 73.39,43.71 74.2,42.9 111.9,42.9 119.1,50.1 126.91,50.1 SV1.2
J_MCLK_R
  Top 0.254: U$2.P$2 22.18,50.38 22,50.2 22,49.5 22.4,49.1 33.6,49.1 | U$1.P$2 33.77,50.38 33.6,50.2 33.6,49.1 | U$4.P$2 43.48,43.52 43.3,43.35 43.3,42.25 | 43.3,42.25 54.9,42.25 | U$3.P$2 55.08,43.52 54.9,43.35 54.9,42.25 | 43.3,42.25 40.45,42.25 33.6,49.1 | R14.2 65.06,43.71 63.4,42.05 55.1,42.05 54.9,42.25
LB_B
  Top 0.254: U6.42 134.3,25.8 129.35,20.85 SV1.26
LB_T
  Bottom 0.254: U5.42 139.8,25.7 144.65,20.85 SV2.25
N$1
  Top 0.254: U7.1 C1.1
N$2
  Top 0.254: U7.3 143.21,65.75 C1.2
N$3
  Top 0.254: U7.4 141.94,66.58 C2.1
N$4
  Top 0.254: U7.5 140.66,65.64 140.3,66 140.3,66.55 C2.2
N$5  (via drill 0.33)
  Top 0.254: U7.2 v144.47,62.23
  Bottom 0.254: v144.47,62.23 147.98,62.23 C3.1
N$6  (via drill 0.33)
  Top 0.254: U7.6 v139.4,62.2
  Bottom 0.254: v139.4,62.2 134.66,62.2 C4.1
N$8
  Top 0.254: U7.13 141.94,59.87 141.3,60.5 134.8,60.5 128.09,67.21 X1.2
N$9
  Top 0.254: X1.3 126.59,73.95 131.75,73.95 138.12,67.58 U7.7
N$11
  Top 0.254: X3.4 83.8,69.6 86.1,71.9 R23.2 R22.1
N$12
  Top 0.254: R4.2 20.6,60.75 R3.1 20.45,61.45 13.72,68.17 13.2,68.7 13.1,68.8 X2.1
N$13
  pour Top (isolate 1.016): 0,38.25 120.75,38.25 120.75,0 0,0
N$14
  Top 0.254: R6.2 34.55,58.2 R5.1 35.4,56.3 35.08,55.98 U$1.P$05
N$15
  Top 0.254: X2.2 15.6,68.3 20.2,63.7 29.8,63.7 32,61.5 32,60.65 R2.1 arc-90 32.2,60.75 R5.2
N$16
  Top 0.254: X3.6 54.9,67.1 56.2,68.4 84.9,68.4 86.1,69.6 R24.2 R21.1
N$17
  Top 0.254: R10.2 41.8,53.9 R9.1 41.75,58.65 35.75,64.65 X3.1
N$18
  Top 0.254: R13.2 44.25,51.35 R10.1 45.1,49.45 44.77,49.12 U$4.P$05
N$19
  Top 0.254: U$3.P$05 56.38,49.12 56.7,49.45 R11.1 56.05,51.25 R12.2
N$20
  Top 0.254: R11.2 56.65,53.85 R8.1 53.15,54.8 51.2,56.75 47.85,56.75 47.8,56.8 46.58,58.02 38.2,66.4 X3.2
N$21
  Top 0.254: X2.4 25.6,73.3 26.9,74.6 61.5,74.6 62.6,75.7 R17.2 R16.1
N$22
  Top 0.254: X2.6 23.2,69.8 23.2,72.5 26.5,75.8 60.3,75.8 62.5,78 R18.2 R15.1
N$25
  Top 0.254: R7.2 22.95,58.2 R4.1 23.8,56.3 23.48,55.98 U$2.P$05
N$27
  Bottom 0.254: R1.1 124,69 124,73.3 124.8,74.1 125.57,74.1 X1.7
N$28  (via drill 0.33)
  Top 0.254: U7.14 143.21,60.59 142.5,61.3 136.9,61.3 v133.3,64.9
  Bottom 0.254: X1.4 122.6,67.3 124.6,65.3 R1.2 132.9,65.3 v133.3,64.9
OE_B
  Top 0.254: U6.44 133.3,29.6 130.6,32.3 126.85,32.3 SV1.15
OE_T
  Bottom 0.254: U5.44 140.8,29.3 143.8,32.3 147.21,32.3 SV2.16
RST
  Top 0.254: SV2.7 145.41,43.71 145.4,43.7 144.7,43.7 136.2,52.2 133.1,52.2 131.3,54 72.03,54 SV4.4 67.83,58.23
RW_B
  Top 0.254: U6.18 139.8,7.2 142.7,4.3 147.15,4.3 SV2.38
RW_T
  Bottom 0.254: U5.18 134.3,7.3 131.3,4.3 126.91,4.3 SV1.37
RXD0
  Top 0.254: U7.12 140.66,56.34 144.4,52.6 147.19,52.6 SV2.2
TXD0
  Top 0.254: U7.10 138.12,56.38 143.17,51.33 SV2.1
UB_B
  Top 0.254: U6.43 133.8,26.8 129.1,22.1 126.89,22.1 SV1.23
UB_T
  Bottom 0.254: U5.43 140.3,26.5 144.7,22.1 147.17,22.1 SV2.24
WF_RXD
  Top 0.254: SV2.8 147.17,45 144.4,45 136.5,52.9 133.4,52.9 131.6,54.7 76.41,54.7 SV4.1
WF_TXD
  Top 0.254: SV2.10 147.23,42.4 145,42.4 135.9,51.5 132.8,51.5 131,53.3 67.65,53.3 SV4.8

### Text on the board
tNames: MAX3232 | Wi Fi | RTC
bNames: CoCo3 FPGA Analog Board - REV02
